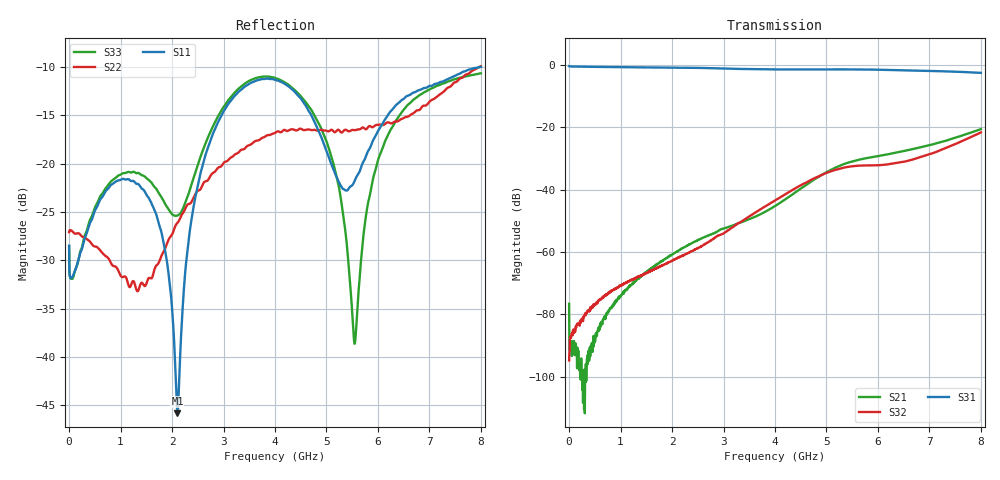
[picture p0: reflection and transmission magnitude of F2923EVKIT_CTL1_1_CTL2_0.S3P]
! Integrated Device Technology
! Corporate Headquarters
! 6024 Silver Creek Valley Road
! San Jose, CA 95138  USA
! Phone:  1-408-284-8200
! Toll Free:  1-800-223-1366
! Webpage:  http://www.idt.com/
! Timing and RF Division
! 515 Groton Road, Suite 102
! Westford, MA 01886-6024
! Device:  F2923
! Description: Constant Impedance Kz SP2T RF Switch
! Frequency:  0.3 MHz to 8 GHz
! Package:  4 mm x 4 mm QFN Plastic Package: 20 pin
! Ports:  3 RF, 3 DC
!  Pin  1  = GND
!  Pin  2  = GND
!  Pin  3  = RF1  = Port 1
!  Pin  4  = GND
!  Pin  5  = GND
!  Pin  6  = GND
!  Pin  7  = GND
!  Pin  8  = RF_COM  = Port 3
!  Pin  9  = GND
!  Pin  10  = GND
!  Pin  11  = GND
!  Pin  12  = GND
!  Pin  13  = RF2  = Port 2
!  Pin  14  = GND
!  Pin  15  = NC
!  Pin  16  = CTL2
!  Pin  17  = CTL1
!  Pin  18  = NC
!  Pin  19  = ModeCTL
!  Pin  20  = VCC
!  EP  = GND
! State:  RF1 On
! Voltage:  VCC  = +3.3 V
!  CTL1  = 3.3 V (Logic HIGH)
!  CTL2  = 0 V (Logic LOW)
! Data:  The device was measured on the F2923 EVKit
!  using a calibrated network analyzer.
!  The results below include the EVKit RF connector and
!		PCB loss effects. The reference plane is at
!  the SMA coaxial interface. Refer to the separate
!  measured thru line.s2p file for connector and PCB loss
!  and effects.
! Misc:
! Date Measured:  2017-8-14
! Date:  2017-8-14  SPJ
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# Hz S dB R 50
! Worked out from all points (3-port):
!   1601 points, 300 kHz to 8 GHz, reference 50 ohm
!   strongest paths, dB at 300 kHz, 2 GHz, 4 GHz, 6 GHz, 8 GHz:
!     S31: -0.3, -0.8, -1.4, -1.5, -2.5
!     S32: -94.7, -62.7, -43.4, -32.1, -21.6
!     S21: -76.6, -60.8, -45.2, -29.2, -20.5
!   lowest |S11| = -45.8 dB at 2.105 GHz (marker M1), VSWR 1.01, Z = 49.7 + j0.376 ohm
!   |S11| at or under -10 dB: start of sweep to end of sweep
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300000  -28.48 -5.6  -90.76 74.5  -0.32 0.1
        -76.55 -51.9  -27.08 178.7  -87.09 165.2
        -0.32 0.1  -94.73 -31.7  -28.55 -6.6
9.302651e8  -21.78 -169.2  -75.68 81.2  -0.63 -100.1
            -75.49 81.5  -30.80 134.6  -71.48 22.6
            -0.63 -100.1  -71.46 23.2  -21.33 -163.0
2.105221e9  -45.81 132.3  -59.69 -14.4  -0.79 134.7
            -59.66 -14.6  -26.13 149.0  -61.94 -39.4
            -0.80 134.7  -61.84 -38.9  -25.37 134.3
3.175181e9  -13.26 111.8  -51.54 -111.4  -1.14 20.4
            -51.48 -110.8  -19.27 88.5  -51.99 -105.4
            -1.15 20.4  -52.03 -105.4  -12.89 92.6
4.00015e9  -11.34 31.7  -45.20 -172.7  -1.37 -66.2
           -45.22 -173.0  -16.83 37.9  -43.41 -179.2
           -1.37 -66.1  -43.42 -179.1  -11.14 14.4
4.995113e9  -18.61 -48.7  -34.41 81.3  -1.32 -172.1
            -34.38 81.2  -16.59 -21.9  -34.57 64.1
            -1.32 -172.1  -34.61 63.9  -17.60 -90.1
5.545092e9  -21.80 -33.9  -30.63 6.5  -1.37 128.2
            -30.69 6.9  -16.54 -50.6  -32.38 -8.6
            -1.37 128.2  -32.36 -8.7  -38.62 133.3
5.86508e9  -18.14 -40.6  -29.49 -34.2  -1.42 93.3
           -29.56 -34.5  -16.17 -67.5  -32.11 -45.8
           -1.42 93.3  -32.16 -45.6  -22.63 14.4
6.785046e9  -12.42 -117.4  -26.54 -139.4  -1.75 -7.3
            -26.51 -139.2  -14.48 -117.8  -29.77 -131.6
            -1.76 -7.4  -29.71 -132.3  -13.00 -88.9
8e9  -10.00 100.8  -20.54 85.1  -2.44 -142.0
     -20.52 84.3  -9.92 144.7  -21.53 105.3
     -2.47 -142.0  -21.58 105.3  -10.66 139.3
